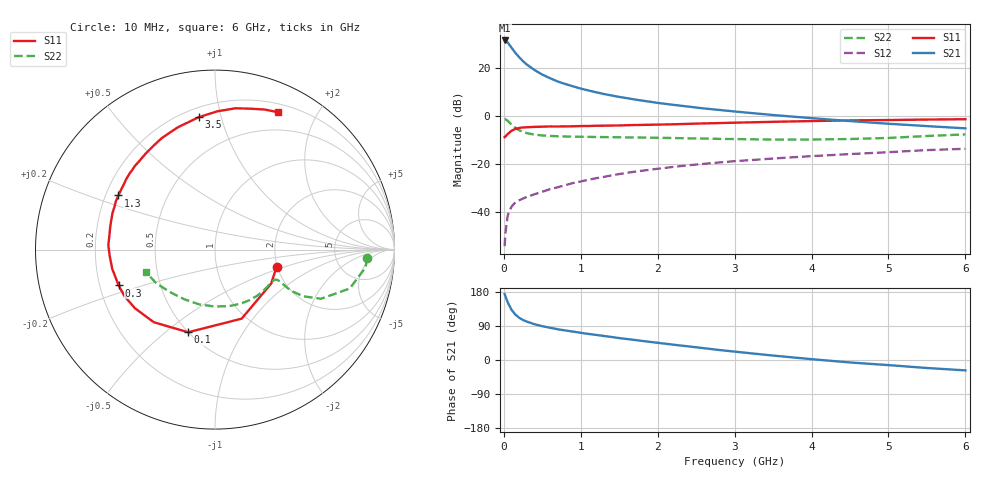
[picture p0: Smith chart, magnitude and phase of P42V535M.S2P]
! SIEMENS Small Signal Semiconductors
! BFP182
! Si NPN RF Bipolar Junction Transistor in SOT143
! VCE = 2.5 V  IC = 35 mA
! Common Emitter S-Parameters:  March  1996
# GHz  S  MA  R  50
!  f  S11  S21  S12  S22
! GHz  MAG  ANG  MAG  ANG  MAG  ANG  MAG  ANG
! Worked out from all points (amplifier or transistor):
!   36 points, 10 MHz to 6 GHz, reference 50 ohm
!   highest |S21| = 31.3 dB at 10 MHz (marker M1)
!   |S21| within 3 dB of that: start of sweep to 99.52 MHz
!   unconditionally stable (mu >= 1): start of sweep to 19.69 MHz; 272.9 MHz to end of sweep
!   at 250 MHz: K = 0.95, MSG = 28.6 dB, |S12| = -34.6 dB
!   at 1.4 GHz: K = 1.65, MAG = 11.9 dB, |S12| = -24.9 dB
!   at 6 GHz: K = 1.14, MAG = 2.0 dB, |S12| = -13.8 dB
!   S11 on the Smith chart (normalised r, x): 10 MHz: 1.98, -0.43; 100 MHz: 0.50, -0.60; 300 MHz: 0.28, -0.17; 1.3 GHz: 0.25, +0.25; 3.5 GHz: 0.26, +0.85; 6 GHz: 0.29, +1.53
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0.01  0.3563 -15.6  36.89 174.0  0.0019 73.1  0.8501 -3.1
0.02  0.3658 -31.1  36.8 168.4  0.0035 72.1  0.8441 -6.8
0.05  0.4125 -68.9  33.52 152.0  0.0083 68.7  0.7814 -16.1
0.1  0.4842 -108.0  26.05 132.4  0.0127 52.9  0.6506 -24.9
0.15  0.5291 -130.1  20.38 119.8  0.0156 48.8  0.556 -27.9
0.2  0.5528 -143.7  16.46 111.4  0.0172 48.6  0.4954 -28.3
0.25  0.5672 -152.8  13.61 105.5  0.0187 47.3  0.4571 -27.9
0.3  0.5725 -159.6  11.58 101.2  0.0202 48.4  0.4313 -27.1
0.4  0.5828 -169.4  8.902 94.3  0.023 51.5  0.4018 -26.1
0.5  0.588 -176.8  7.165 89.2  0.0259 52.7  0.386 -25.9
0.6  0.5949 177.5  6.03 85.0  0.0293 55.4  0.3775 -26.3
0.7  0.5934 172.5  5.153 81.2  0.0321 56.8  0.3712 -27.1
0.8  0.5968 168.3  4.552 77.9  0.0356 58.1  0.3672 -28.2
1.1  0.6084 157.3  3.346 68.8  0.0461 59.0  0.36 -32.7
1.3  0.6168 150.7  2.823 63.4  0.0528 58.9  0.3568 -36.2
1.7  0.637 138.4  2.17 52.9  0.0678 57.5  0.3502 -44.0
2.2  0.6603 125.6  1.68 40.5  0.0852 53.9  0.3417 -55.2
2.8  0.6993 110.9  1.315 26.4  0.1057 48.6  0.3277 -70.3
3.5  0.7429 97.1  1.029 11.7  0.1276 42.1  0.3169 -90.7
4.5  0.7957 81.7  0.77 -6.5  0.1578 33.0  0.3253 -121.5
5.5  0.828 70.5  0.605 -21.1  0.1912 23.6  0.376 -149.6
6  0.8426 65.2  0.543 -27.4  0.2034 18.0  0.4062 -162.1
